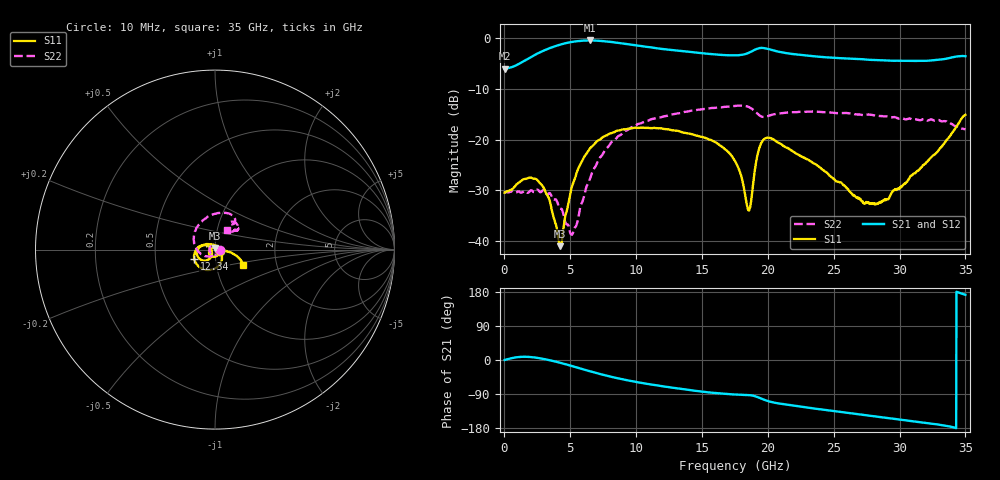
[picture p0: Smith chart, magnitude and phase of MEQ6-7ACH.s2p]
! MARKI MICROWAVE INC.
! Email:  support@markimicrowave.com  Phone:  408-778-4200
! Model Number:  MEQ6-7ACH  Date:  6/18
! Filename:		MEQ6-7ACH.S2P  Version: 1.0
! Description:  2-port S-parameter data for chip equalizer
! Features:		Low Insertion Loss, Excellent Return Loss
! Frequency Measured: 	10 MHz to 35 GHz
!S2P File: Measurements: S11, S21, S12, S22:
# Hz S  dB  R 50
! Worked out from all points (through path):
!   1601 points, 10 MHz to 35 GHz, reference 50 ohm
!   highest |S21| = -0.47 dB at 6.505 GHz (marker M1); lowest = -6.1 dB at 10 MHz (marker M2)
!   group delay of S21, straight-line fit = 15.4 ps
!   lowest |S11| = -41.0 dB at 4.209 GHz (marker M3), VSWR 1.02, Z = 50.2 + j0.871 ohm
!   |S11| at or under -10 dB: start of sweep to end of sweep
!   |S22| runs from -38.8 to -13.3 dB; largest |S21 - S12| = 0.0074
!   S11 on the Smith chart (normalised r, x): 10 MHz: 1.06, -0.01; 12.34 GHz: 0.79, -0.08; 35 GHz: 1.34, -0.23
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1e7  -30.47 -11.2  -6.06 0.1  -6.03 0.6  -30.47 -3.2
1.497075e9  -27.80 -101.3  -4.49 8.6  -4.49 8.5  -30.15 -101.8
2.503038e9  -28.01 -146.8  -3.05 5.6  -3.05 5.7  -29.89 -165.6
3.355919e9  -31.52 176.3  -2.06 -0.0  -2.06 0.0  -30.64 142.7
4.2088e9  -41.03 77.7  -1.31 -7.1  -1.31 -7.1  -33.59 94.7
5.105419e9  -29.40 -22.9  -0.76 -15.7  -0.76 -15.7  -38.78 3.7
5.848956e9  -24.50 -49.4  -0.53 -23.3  -0.53 -23.2  -32.63 -79.7
6.505019e9  -21.72 -67.7  -0.47 -29.9  -0.47 -29.8  -27.70 -119.1
8.23265e9  -18.65 -104.9  -0.81 -45.4  -0.79 -45.4  -20.27 -174.9
1.168791e10  -17.78 -149.9  -2.05 -67.8  -2.03 -67.7  -15.65 123.7
1.234398e10  -17.97 -156.7  -2.25 -71.0  -2.23 -71.0  -15.34 116.4
1.577737e10  -20.23 173.4  -3.18 -86.4  -3.14 -86.4  -13.76 85.2
1.7505e10  -24.21 156.4  -3.41 -91.2  -3.39 -91.2  -13.38 71.2
1.853283e10  -33.98 -166.5  -2.92 -92.4  -2.90 -92.3  -13.57 59.2
1.870778e10  -32.60 -135.2  -2.71 -93.1  -2.69 -93.0  -13.81 56.8
1.92545e10  -22.58 -126.7  -2.05 -98.4  -2.00 -98.3  -15.01 54.0
1.977935e10  -19.81 -153.3  -2.01 -105.8  -1.94 -105.8  -15.53 59.2
2.334396e10  -24.44 151.1  -3.55 -127.2  -3.51 -127.1  -14.48 51.7
2.725846e10  -32.57 93.6  -4.18 -145.2  -4.16 -145.1  -15.17 43.2
2.918291e10  -31.60 29.5  -4.43 -153.5  -4.39 -153.9  -15.50 41.5
3.357853e10  -20.10 -12.3  -4.05 -173.9  -3.98 -173.9  -16.45 44.7
3.5e10  -15.12 -28.5  -3.57 172.0  -3.55 172.4  -17.99 57.8
